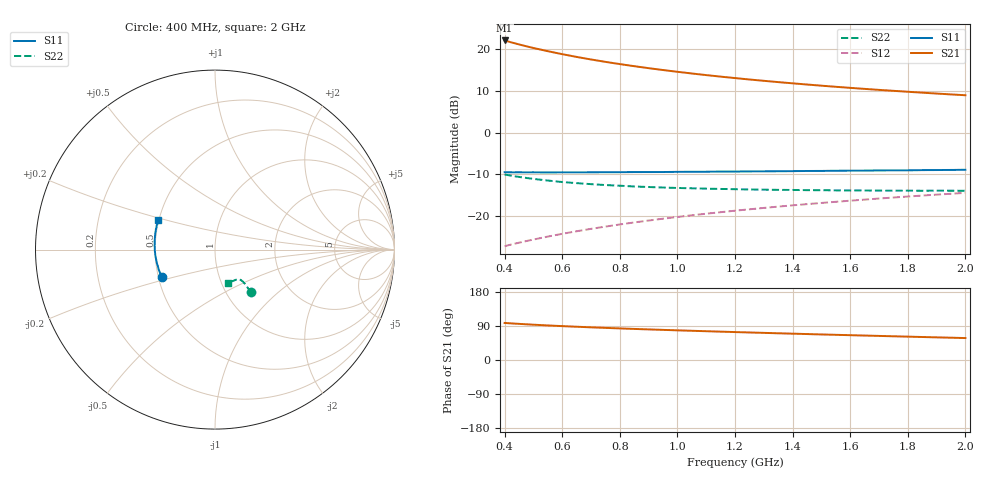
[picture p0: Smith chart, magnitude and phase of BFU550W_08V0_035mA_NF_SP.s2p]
! Filename:  P:\Prog\Test\Noise\ATS_data\Testdata_Net\06 Compressed Noise after Statistics\BFU550W_APM2013_11_D05_08p0V_035mA_NF_CM01_D.sf
! Date/Time: Tue 26/Mar/2013 16:25:25
! BFU550W_APM2013_11_D05_08p0V_1to35mA_NF_CM01_Bias9_R.sf
! Noise Parameter Data File
! BFU550W_APM2013_11_D05_08p0V_1to35mA_NF_CM01
! Date/time: Mon Mar 25 14:39:45 2013
! VAR V_out= 8.000000
! VAR I_out= 34.990000
! VAR V_in= 0.780600
! VAR I_in= 0.349300
! Device data file deembeded for feedlines and parallel
! Original file: \06 Compressed Noise after Statistics\BFU550W_APM2013_11_D05_08p0V_035mA_NF_CM01_R.sf
! Feed-files: PR019V01_070313_Feed1.s2p, PR019V01_070313_Feed2.s2p
! Parallel-file: PR019V01_070313_Par.s2p
# MHz S MA R 50
!  Freq-MHz  S11-mag  S11-arg  S21-mag  S21-arg  S12-mag  S12-arg  S22-mag  S22-arg
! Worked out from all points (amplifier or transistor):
!   37 points, 400 MHz to 2 GHz, reference 50 ohm
!   highest |S21| = 22.2 dB at 400 MHz (marker M1)
!   |S21| within 3 dB of that: start of sweep to 579.4 MHz
!   unconditionally stable (mu >= 1): 877.2 MHz to end of sweep
!   at 500 MHz: K = 0.94, MSG = 23.0 dB, |S12| = -25.7 dB
!   at 1.1 GHz: K = 1.01, MAG = 16.1 dB, |S12| = -19.5 dB
!   at 2 GHz: K = 1.00, MAG = 11.6 dB, |S12| = -14.5 dB
!   lowest NFmin = 1.26 dB at 440 MHz
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400  0.3333 -152.5  12.83 97.8  0.04305 70.1  0.3129 -49.8
433  0.3326 -155.6  11.92 96.2  0.04591 70.5  0.2994 -49.6
460  0.3329 -157.7  11.26 94.9  0.04825 71.0  0.2898 -49.5
480  0.3326 -159.3  10.82 94.0  0.04999 71.2  0.2835 -49.5
500  0.333 -160.8  10.42 93.2  0.05171 71.4  0.2774 -49.3
550  0.3313 -164.1  9.536 91.2  0.05615 71.8  0.2651 -49.1
600  0.3327 -167.0  8.781 89.4  0.06061 72.2  0.2544 -48.9
650  0.3322 -169.6  8.135 87.8  0.06507 72.4  0.2467 -48.9
700  0.3331 -172.1  7.577 86.2  0.06956 72.6  0.2398 -48.9
750  0.3338 -174.2  7.094 84.8  0.07403 72.7  0.234 -49.0
800  0.3342 -176.4  6.669 83.3  0.07851 72.8  0.2295 -49.4
850  0.3352 -178.4  6.293 82.0  0.08302 72.8  0.2249 -49.4
900  0.3354 180.0  5.958 80.7  0.08756 72.8  0.2215 -49.8
950  0.3356 178.2  5.657 79.5  0.09213 72.7  0.2185 -50.1
1050  0.3377 175.0  5.141 77.1  0.1013 72.5  0.2138 -51.2
1150  0.3403 171.9  4.713 74.8  0.1103 72.1  0.21 -52.4
1200  0.3401 170.6  4.529 73.7  0.115 71.9  0.2086 -53.1
1350  0.3428 166.7  4.05 70.5  0.1288 71.2  0.2047 -55.1
1500  0.3459 162.9  3.668 67.4  0.1425 70.4  0.2029 -57.8
1650  0.3491 159.3  3.356 64.5  0.1563 69.4  0.2012 -60.4
1750  0.3513 157.3  3.181 62.6  0.1656 68.8  0.2001 -62.4
2000  0.3571 152.0  2.815 57.9  0.1885 66.9  0.1999 -68.0
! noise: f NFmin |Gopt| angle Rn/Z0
400  1.272  0.3628  -171.7  0.0796
460  1.289  0.3848  -170.8  0.0705
600  1.318  0.3697  -165.8  0.0803
800  1.336  0.3952  -162.6  0.0767
1000  1.364  0.3997  -158.6  0.0806
1200  1.392  0.4045  -153  0.09
1400  1.411  0.4198  -149.1  0.0959
1600  1.442  0.4274  -146.6  0.1001
1800  1.47  0.4335  -141.2  0.1162
2000  1.493  0.4425  -138.7  0.1256
